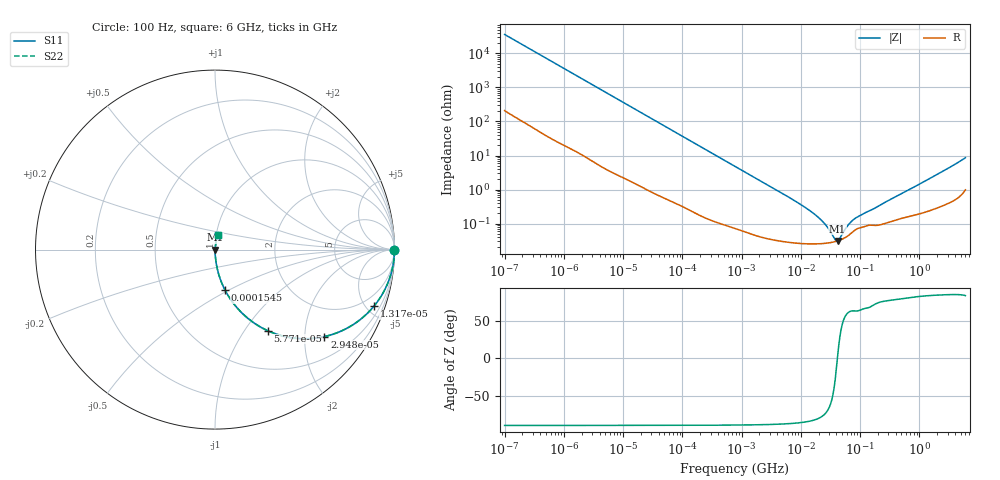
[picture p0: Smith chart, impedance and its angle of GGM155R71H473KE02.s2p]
!Murata Part Number: GGM155R71H473KE02
!These Parameters are Measured in Series Mode Connection
!Data Generated on Mar 13, 2026
!  o--ll--o
!Port1  Port2
!  o------o
!Operation Temp=25[degC], DC Bias Voltage=0[V]
!Freq. Start=100[Hz] Stop=6[GHz] 401[Steps]
# Hz S RI R 50
!Freq.(Hz) S11(Real) S11(Imag) S21(Real) S21(Imag) S12(Real) S12(Imag) S22(Real) S22(Imag)
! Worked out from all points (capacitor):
!   401 points, 100 Hz to 6 GHz, reference 50 ohm
!   read as one part in series: C = 43.9 nF near 109 Hz
!   lowest |Z| = 30.8 mohm at 41.66 MHz (marker M1)
!   series resonance near 41.48 MHz, so ESL is about 340 pH
!   S11 on the Smith chart (normalised r, x): 100 Hz: open; 13.17 kHz: 1.04, -5.59; 29.48 kHz: 1.02, -2.50; 57.71 kHz: 1.01, -1.28; 154.5 kHz: 1.00, -0.48; 6 GHz: 1.02, +0.17
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100  1 -0.00276  2.36e-05 0.00276  2.36e-05 0.00276  1 -0.00276
2008  0.9967 -0.0547  0.00332 0.0547  0.00332 0.0547  0.9967 -0.0547
5378  0.9782 -0.1433  0.0218 0.1433  0.0218 0.1433  0.9782 -0.1433
13169  0.885 -0.3159  0.115 0.3159  0.115 0.3159  0.885 -0.3159
19704  0.7763 -0.4135  0.2237 0.4135  0.2237 0.4135  0.7763 -0.4135
29482  0.61 -0.4844  0.39 0.4844  0.39 0.4844  0.61 -0.4844
40335  0.4569 -0.4946  0.5431 0.4946  0.5431 0.4946  0.4569 -0.4946
57709  0.2931 -0.4513  0.7069 0.4513  0.7069 0.4513  0.2931 -0.4513
90302  0.1466 -0.3495  0.8534 0.3495  0.8534 0.3495  0.1466 -0.3495
154540  0.0566 -0.2267  0.9434 0.2267  0.9434 0.2267  0.0566 -0.2267
316350  0.0149 -0.1161  0.9851 0.1161  0.9851 0.1161  0.0149 -0.1161
774597  0.00305 -0.0483  0.9969 0.0483  0.9969 0.0483  0.00305 -0.0483
6353432  0.000313 -0.00585  0.9997 0.00585  0.9997 0.00585  0.000313 -0.00585
1.555665e7  0.000256 -0.00211  0.9997 0.00211  0.9997 0.00211  0.000256 -0.00211
2.434276e7  0.00026 -0.00103  0.9997 0.00103  0.9997 0.00103  0.00026 -0.00103
3.64232e7  0.000289 -0.000241  0.9997 0.000241  0.9997 0.000241  0.000289 -0.000241
4.165952e7  0.000307 8.1e-06  0.9997 -8.1e-06  0.9997 -8.1e-06  0.000307 8.1e-06
4.556224e7  0.000324 0.000174  0.9997 -0.000174  0.9997 -0.000174  0.000324 0.000174
6.233367e7  0.000435 0.000767  0.9996 -0.000767  0.9996 -0.000767  0.000435 0.000767
7.797396e7  0.000597 0.00117  0.9994 -0.00117  0.9994 -0.00117  0.000597 0.00117
3.124326e8  0.00113 0.00479  0.9989 -0.00479  0.9989 -0.00479  0.00113 0.00479
6e9  0.0167 0.0833  0.9833 -0.0833  0.9833 -0.0833  0.0167 0.0833
